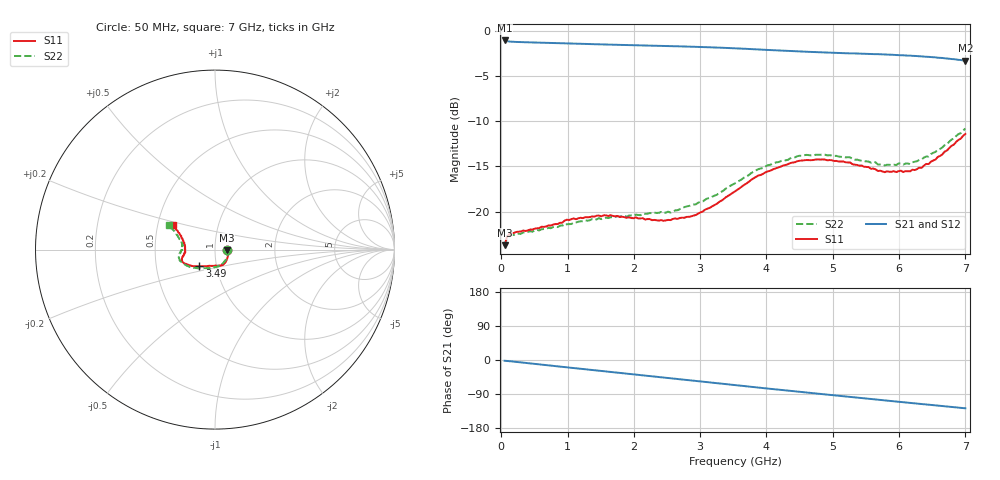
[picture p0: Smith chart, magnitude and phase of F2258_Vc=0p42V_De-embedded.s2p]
! Integrated Device Technology
! Corporate Headquarters
! 6024 Silver Creek Valley Road
! San Jose, CA 95138  USA
! Phone:  1-408-284-8200
! Toll Free:  1-800-223-1366
! Webpage:  http://www.idt.com/
! Timing and RF Division
! 515 Groton Road, Suite 102
! Westford, MA 01886-6024
! Device:  F2258
! Description: Voltage Variable RF Attenuator
! Frequency:  50.0 -  6000.00 MHz
! Package:  3x3 mm Thin QFN Plastic Package: 16 pin
! Ports:  2 RF, 2 DC
!  Pin  1  = NC
!  Pin  2  = NC
!  Pin  3  = RF2  = Port 2
!  Pin  4  = GND
!  Pin  5  = Vdd
!  Pin  6  = NC
!  Pin  7  = VCTRL
!  Pin  8  = NC
!  Pin  9  = GND
!  Pin 10  = RF1  = Port 1
!  Pin 11  = NC
!  Pin 12  = NC
!  Pin 13  = NC
!  Pin 14  = NC
!  Pin 15  = NC
!  Pin 16  = NC
! Vcntrl:  0.420 Volts
! Vdd:  +3.300 Volts
! Current:  1.095 mA
! Data:  The device was measured on a the F2258 evaluation board which has
!  individual transmission lines to the RF pins.  Data was collected
!  using a calibrated network analyzer.  The evaluation board was
!  de-embedded using a TRL calibration technique.
!  The reference plane is the edge of the package pin.
! Misc:  SN 10
!  Action Tracker AT0285
! Date Measured:  2014-12-10
! Date:  2016-01-13  MJV
! Note:
!  Integrated Device Technology supplies this data as a sample of measured
!  data at the package pin for this product.  Your particular data for this
!  product may vary.
!  Data was taken at 25 degrees C.
!  Integrated Device Technology reserves the right to change this data at anytime.
!Freq_(GHz)  S11M_(dB)  S11P_(deg)  S21M_(dB)  S21P_(deg)  S12M_(dB)  S12P_(deg)  S22M_(dB)  S22P_(deg)
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# GHz S dB R 50
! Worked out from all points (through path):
!   201 points, 50 MHz to 7 GHz, reference 50 ohm
!   highest |S21| = -1.03 dB at 50 MHz (marker M1); lowest = -3.3 dB at 7 GHz (marker M2)
!   group delay of S21, straight-line fit = 50.5 ps
!   lowest |S11| = -23.7 dB at 50 MHz (marker M3), VSWR 1.14, Z = 56.9 - j0.428 ohm
!   |S11| at or under -10 dB: start of sweep to end of sweep
!   |S22| runs from -23.8 to -10.8 dB; largest |S21 - S12| = 0.00033
!   S11 on the Smith chart (normalised r, x): 50 MHz: 1.14, -0.01; 3.49 GHz: 0.83, -0.16; 7 GHz: 0.60, +0.18
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0.05  -23.74 -3.3  -1.03 -2.0  -1.03 -2.0  -23.83 -3.1
0.08475  -22.81 -5.4  -1.11 -2.5  -1.11 -2.5  -22.93 -5.2
0.15425  -22.35 -8.4  -1.17 -3.6  -1.17 -3.7  -22.57 -8.9
0.71025  -21.54 -34.2  -1.30 -14.1  -1.30 -14.1  -21.80 -36.8
0.98825  -20.90 -47.4  -1.36 -19.4  -1.36 -19.4  -21.40 -52.3
1.2315  -20.72 -55.3  -1.41 -23.8  -1.41 -23.8  -21.06 -61.2
1.6485  -20.40 -66.7  -1.50 -31.4  -1.50 -31.4  -20.63 -74.3
2.37825  -20.99 -87.1  -1.63 -44.8  -1.63 -44.8  -20.13 -92.4
2.552  -20.94 -92.9  -1.66 -48.0  -1.66 -48.0  -20.11 -97.7
2.93425  -20.38 -109.7  -1.74 -55.1  -1.74 -55.1  -19.19 -111.2
3.49025  -17.91 -132.9  -1.89 -65.6  -1.89 -65.6  -17.00 -132.7
3.525  -17.77 -133.8  -1.90 -66.2  -1.90 -66.2  -16.86 -134.2
4.0115  -15.56 -148.4  -2.08 -75.2  -2.08 -75.2  -14.88 -149.9
4.46325  -14.42 -157.2  -2.24 -83.4  -2.24 -83.4  -13.86 -161.2
4.7065  -14.28 -160.5  -2.31 -87.7  -2.32 -87.7  -13.76 -165.5
5.2625  -14.56 -167.3  -2.47 -97.4  -2.47 -97.4  -13.99 -173.6
5.6795  -15.50 -173.8  -2.55 -104.6  -2.55 -104.6  -14.78 -179.2
5.85325  -15.58 -177.9  -2.61 -107.8  -2.61 -107.8  -14.81 176.2
6.166  -15.54 174.1  -2.71 -113.4  -2.72 -113.3  -14.73 170.2
6.33975  -15.15 167.5  -2.80 -116.5  -2.80 -116.5  -14.21 165.7
6.722  -13.23 155.3  -3.03 -123.1  -3.03 -123.1  -12.55 156.6
7  -11.39 149.5  -3.27 -127.4  -3.28 -127.4  -10.80 151.6
